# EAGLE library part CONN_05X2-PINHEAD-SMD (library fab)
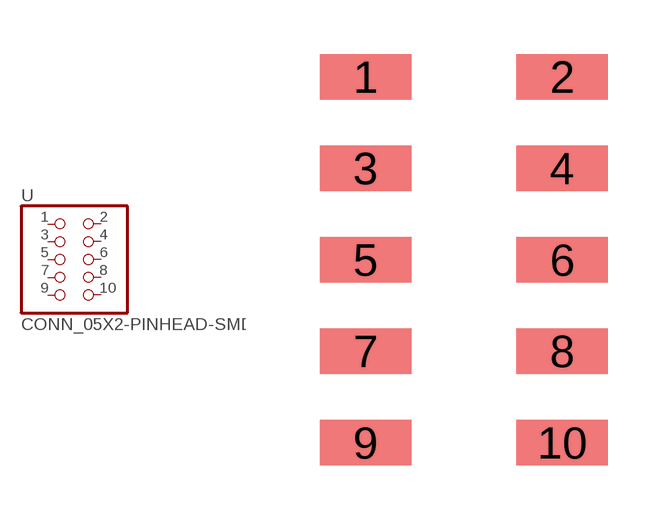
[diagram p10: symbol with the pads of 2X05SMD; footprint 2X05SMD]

Designator prefix -

## CONN_05X2-PINHEAD-SMD  [2X05SMD]
1  1  pas
2  2  pas
3  3  pas
4  4  pas
5  5  pas
6  6  pas
7  7  pas
8  8  pas
9  9  pas
10  10  pas

## Footprint 2X05SMD (pad centres in mm)
smd 2.54 x 1.27: 1 -2.54,2.54; 2 2.92,2.54; 3 -2.54,0; 4 2.92,0; 5 -2.54,-2.54; 6 2.92,-2.54; 7 -2.54,-5.08; 8 2.92,-5.08; 9 -2.54,-7.62; 10 2.92,-7.62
